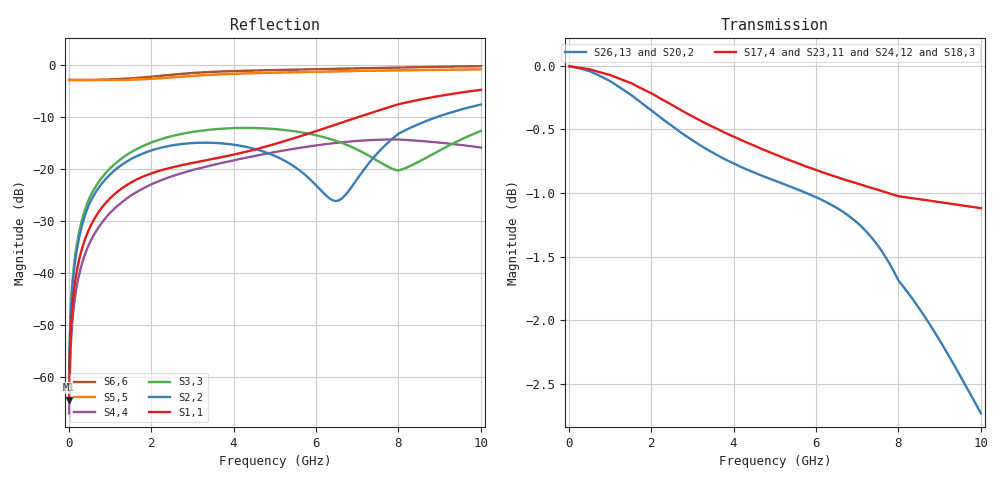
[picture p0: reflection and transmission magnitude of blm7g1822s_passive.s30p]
! Created Wed May 20 10:15:17 2015
! 30 Port Network Data from SP1.SP block
! freq  magS1_1  angS1_1  magS1_2  angS1_2  magS1_3  angS1_3  magS1_4  angS1_4
!  magS1_5  angS1_5  magS1_6  angS1_6  magS1_7  angS1_7  magS1_8  angS1_8
!  magS1_9  angS1_9  magS1_10  angS1_10  magS1_11  angS1_11  magS1_12  angS1_12
!  magS1_13  angS1_13  magS1_14  angS1_14  magS1_15  angS1_15  magS1_16  angS1_16
!  magS1_17  angS1_17  magS1_18  angS1_18  magS1_19  angS1_19  magS1_20  angS1_20
!  magS1_21  angS1_21  magS1_22  angS1_22  magS1_23  angS1_23  magS1_24  angS1_24
!  magS1_25  angS1_25  magS1_26  angS1_26  magS1_27  angS1_27  magS1_28  angS1_28
!  magS1_29  angS1_29  magS1_30  angS1_30
!  magS2_1  angS2_1  magS2_2  angS2_2
!  magS2_3  angS2_3  magS2_4  angS2_4  magS2_5  angS2_5  magS2_6  angS2_6
!  magS2_7  angS2_7  magS2_8  angS2_8  magS2_9  angS2_9  magS2_10  angS2_10
!  magS2_11  angS2_11  magS2_12  angS2_12  magS2_13  angS2_13  magS2_14  angS2_14
!  magS2_15  angS2_15  magS2_16  angS2_16  magS2_17  angS2_17  magS2_18  angS2_18
!  magS2_19  angS2_19  magS2_20  angS2_20  magS2_21  angS2_21  magS2_22  angS2_22
!  magS2_23  angS2_23  magS2_24  angS2_24  magS2_25  angS2_25  magS2_26  angS2_26
!  magS2_27  angS2_27  magS2_28  angS2_28  magS2_29  angS2_29  magS2_30  angS2_30
!  magS3_1  angS3_1  magS3_2  angS3_2  magS3_3  angS3_3  magS3_4  angS3_4
!  magS3_5  angS3_5  magS3_6  angS3_6  magS3_7  angS3_7  magS3_8  angS3_8
!  magS3_9  angS3_9  magS3_10  angS3_10  magS3_11  angS3_11  magS3_12  angS3_12
!  magS3_13  angS3_13  magS3_14  angS3_14  magS3_15  angS3_15  magS3_16  angS3_16
!  magS3_17  angS3_17  magS3_18  angS3_18  magS3_19  angS3_19  magS3_20  angS3_20
!  magS3_21  angS3_21  magS3_22  angS3_22  magS3_23  angS3_23  magS3_24  angS3_24
!  magS3_25  angS3_25  magS3_26  angS3_26  magS3_27  angS3_27  magS3_28  angS3_28
!  magS3_29  angS3_29  magS3_30  angS3_30
!  magS4_1  angS4_1  magS4_2  angS4_2
!  magS4_3  angS4_3  magS4_4  angS4_4  magS4_5  angS4_5  magS4_6  angS4_6
!  magS4_7  angS4_7  magS4_8  angS4_8  magS4_9  angS4_9  magS4_10  angS4_10
!  magS4_11  angS4_11  magS4_12  angS4_12  magS4_13  angS4_13  magS4_14  angS4_14
!  magS4_15  angS4_15  magS4_16  angS4_16  magS4_17  angS4_17  magS4_18  angS4_18
!  magS4_19  angS4_19  magS4_20  angS4_20  magS4_21  angS4_21  magS4_22  angS4_22
!  magS4_23  angS4_23  magS4_24  angS4_24  magS4_25  angS4_25  magS4_26  angS4_26
!  magS4_27  angS4_27  magS4_28  angS4_28  magS4_29  angS4_29  magS4_30  angS4_30
!  magS5_1  angS5_1  magS5_2  angS5_2  magS5_3  angS5_3  magS5_4  angS5_4
!  magS5_5  angS5_5  magS5_6  angS5_6  magS5_7  angS5_7  magS5_8  angS5_8
!  magS5_9  angS5_9  magS5_10  angS5_10  magS5_11  angS5_11  magS5_12  angS5_12
!  magS5_13  angS5_13  magS5_14  angS5_14  magS5_15  angS5_15  magS5_16  angS5_16
!  magS5_17  angS5_17  magS5_18  angS5_18  magS5_19  angS5_19  magS5_20  angS5_20
!  magS5_21  angS5_21  magS5_22  angS5_22  magS5_23  angS5_23  magS5_24  angS5_24
!  magS5_25  angS5_25  magS5_26  angS5_26  magS5_27  angS5_27  magS5_28  angS5_28
!  magS5_29  angS5_29  magS5_30  angS5_30
!  magS6_1  angS6_1  magS6_2  angS6_2
!  magS6_3  angS6_3  magS6_4  angS6_4  magS6_5  angS6_5  magS6_6  angS6_6
!  magS6_7  angS6_7  magS6_8  angS6_8  magS6_9  angS6_9  magS6_10  angS6_10
!  magS6_11  angS6_11  magS6_12  angS6_12  magS6_13  angS6_13  magS6_14  angS6_14
!  magS6_15  angS6_15  magS6_16  angS6_16  magS6_17  angS6_17  magS6_18  angS6_18
!  magS6_19  angS6_19  magS6_20  angS6_20  magS6_21  angS6_21  magS6_22  angS6_22
!  magS7_29  angS7_29  magS7_30  angS7_30
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# ghz S ma R 50
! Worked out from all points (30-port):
!   1000 points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, 10 MHz to 10 GHz, reference 50 ohm
!   strongest paths, dB at 10 MHz, 2.51 GHz, 5.01 GHz, 7.51 GHz, 10 GHz:
!     S17,4: 0.0, -0.3, -0.7, -1.0, -1.1
!     S23,11: 0.0, -0.3, -0.7, -1.0, -1.1
!     S26,13: 0.0, -0.5, -0.9, -1.4, -2.7
!     S20,2: 0.0, -0.5, -0.9, -1.4, -2.7
!     S24,12: 0.0, -0.5, -0.9, -1.0, -1.7
!     S18,3: 0.0, -0.5, -0.9, -1.0, -1.7
!   lowest |S11| = -64.3 dB at 10 MHz (marker M1), VSWR 1.00, Z = 50 + j0.0563 ohm
!   |S11| at or under -10 dB: start of sweep to 7.045 GHz
